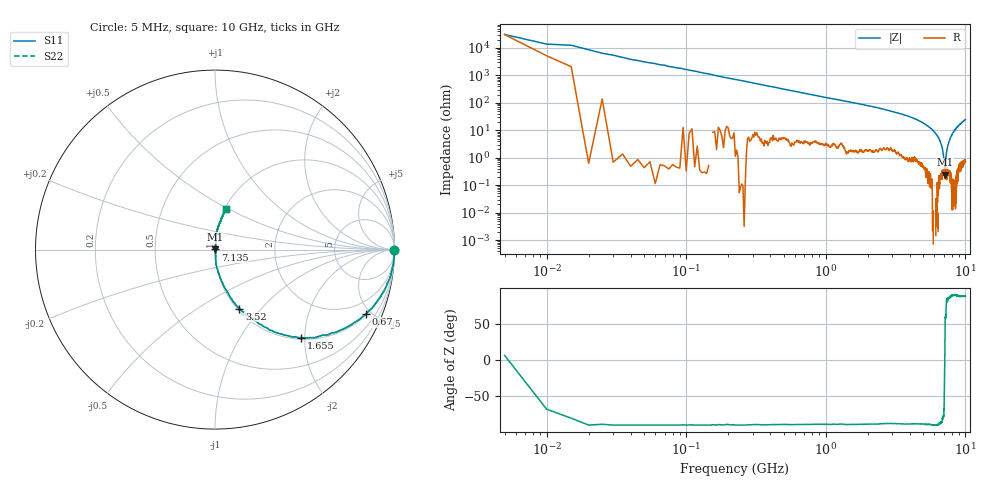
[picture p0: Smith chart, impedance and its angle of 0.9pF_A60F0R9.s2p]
! Amotech Co.,Ltd.
! http://www.amotech.co.kr/
! Part Number: A60F0R9
! These Parameters are Measured in Series Mode Connection
! Operation Temp=25[degC], DC Bias Voltage=0[V]
! Freq. Start=5[MHz] Stop=10[GHz], 2000[Steps]
! Date: Monday, July 20, 2020, 03:12:27
# GHZ S RI R 50.000000
!Freq.(Hz) S11(Real) S11(Imag) S21(Real) S21(Imag) S12(Real) S12(Imag) S22(Real) S22(Imag)
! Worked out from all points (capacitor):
!   2000 points, 5 MHz to 10 GHz, reference 50 ohm
!   read as one part in series: C = 992 fF near 55 MHz
!   lowest |Z| = 242 mohm at 7.15 GHz (marker M1)
!   series resonance near 7.123 GHz, so ESL is about 500 pH
!   S11 on the Smith chart (normalised r, x): 5 MHz: open; 670 MHz: 1.08, -4.67; 1.655 GHz: 1.04, -1.92; 3.52 GHz: 1.02, -0.77; 7.135 GHz: 1.00, +0.00; 10 GHz: 1.02, +0.49
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0.005  0.9968 0.000358  0.00322 -0.000358  0.00322 -0.000358  0.9968 0.000358
0.075  0.9977 -0.0476  0.00228 0.0476  0.00228 0.0476  0.9977 -0.0476
0.175  0.9868 -0.1088  0.0132 0.1088  0.0132 0.1088  0.9868 -0.1088
0.365  0.9475 -0.218  0.0525 0.218  0.0525 0.218  0.9475 -0.218
0.67  0.8412 -0.3576  0.1588 0.3576  0.1588 0.3576  0.8412 -0.3576
1.09  0.6705 -0.4612  0.3295 0.4612  0.3295 0.4612  0.6705 -0.4612
1.655  0.4805 -0.4904  0.5195 0.4904  0.5195 0.4904  0.4805 -0.4904
1.675  0.4753 -0.491  0.5247 0.491  0.5247 0.491  0.4753 -0.491
3.34  0.1547 -0.3445  0.8453 0.3445  0.8453 0.3445  0.1547 -0.3445
3.52  0.1355 -0.3284  0.8645 0.3284  0.8645 0.3284  0.1355 -0.3284
5.005  0.0359 -0.1734  0.9641 0.1734  0.9641 0.1734  0.0359 -0.1734
5.925  0.00858 -0.0944  0.9914 0.0944  0.9914 0.0944  0.00858 -0.0944
6.67  0.00331 -0.0334  0.9967 0.0334  0.9967 0.0334  0.00331 -0.0334
6.84  0.00377 -0.0215  0.9962 0.0215  0.9962 0.0215  0.00377 -0.0215
6.98  0.00256 -0.0111  0.9974 0.0111  0.9974 0.0111  0.00256 -0.0111
7.135  0.00249 0.000669  0.9975 -0.000669  0.9975 -0.000669  0.00249 0.000669
7.15  0.00185 0.00155  0.9981 -0.00155  0.9981 -0.00155  0.00185 0.00155
7.295  0.0034 0.013  0.9966 -0.013  0.9966 -0.013  0.0034 0.013
7.5  0.00311 0.0287  0.9969 -0.0287  0.9969 -0.0287  0.00311 0.0287
7.94  0.00522 0.0648  0.9948 -0.0648  0.9948 -0.0648  0.00522 0.0648
8.335  0.00914 0.0978  0.9909 -0.0978  0.9909 -0.0978  0.00914 0.0978
10  0.0639 0.2287  0.9361 -0.2287  0.9361 -0.2287  0.0639 0.2287
